FUNCTION FC 101 : VOID
TITLE =
VERSION : 0.1

BEGIN
NETWORK
TITLE =
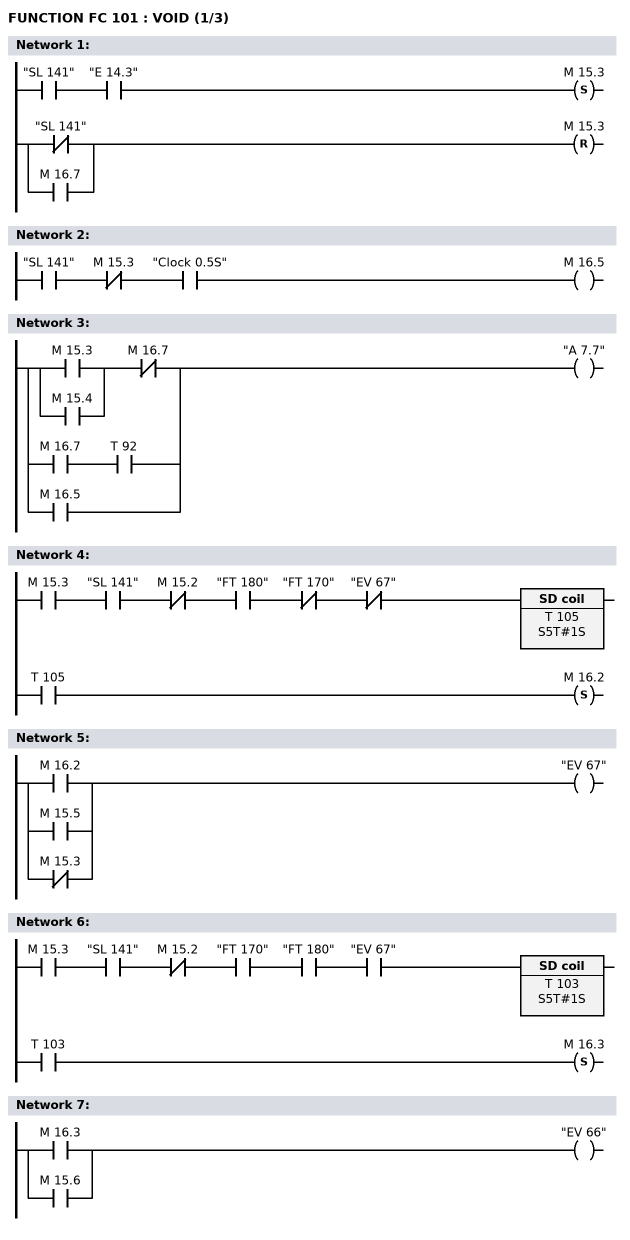
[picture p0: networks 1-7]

      U     "SL 141";
      U     "E      14.3";
      S     M     15.3;
      UN    "SL 141";
      O     M     16.7;
      R     M     15.3;
NETWORK
TITLE =

      U     "SL 141";
      UN    M     15.3;
      U     "Clock 0.5S";
      =     M     16.5;


NETWORK
TITLE =

      U     M     15.3;
      O     M     15.4;
      UN    M     16.7;
      O(    ;
      U     M     16.7;
      U     T     92;
      )     ;
      O     M     16.5;
      =     "A       7.7";
NETWORK
TITLE =

      U     M     15.3;
      U     "SL 141";
      UN    M     15.2;
      U     "FT 180";
      UN    "FT 170";
      UN    "EV 67";
      L     S5T#1S;
      SE    T    105;
      U     T    105;
      S     M     16.2;
NETWORK
TITLE =

      O     M     16.2;
      O     M     15.5;
      ON    M     15.3;
      =     "EV 67";
NETWORK
TITLE =

      U     M     15.3;
      U     "SL 141";
      UN    M     15.2;
      U     "FT 170";
      U     "FT 180";
      U     "EV 67";
      L     S5T#1S;
      SE    T    103;
      U     T    103;
      S     M     16.3;
NETWORK
TITLE =

      O     M     16.3;
      O     M     15.6;
      =     "EV 66";
NETWORK
TITLE =
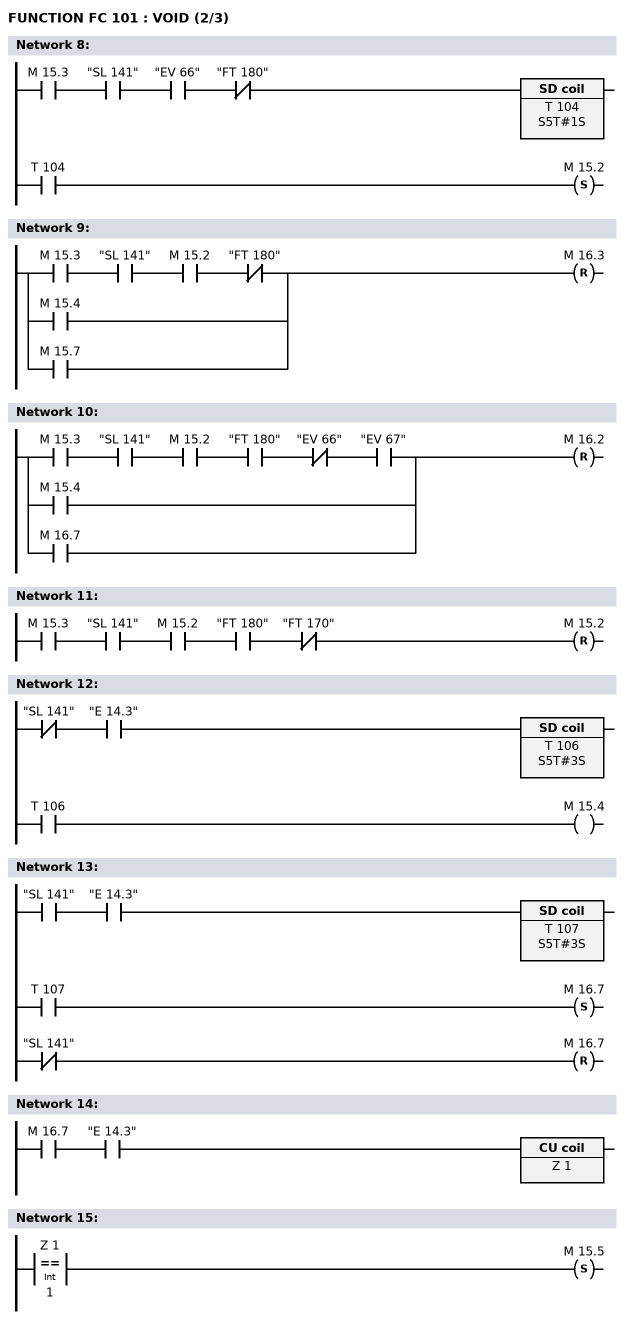
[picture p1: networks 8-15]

      U     M     15.3;
      U     "SL 141";
      U     "EV 66";
      UN    "FT 180";
      L     S5T#1S;
      SE    T    104;
      U     T    104;
      S     M     15.2;
NETWORK
TITLE =

      U     M     15.3;
      U     "SL 141";
      U     M     15.2;
      UN    "FT 180";
      O     M     15.4;
      O     M     15.7;
      R     M     16.3;
NETWORK
TITLE =

      U     M     15.3;
      U     "SL 141";
      U     M     15.2;
      U     "FT 180";
      UN    "EV 66";
      U     "EV 67";
      O     M     15.4;
      O     M     16.7;
      R     M     16.2;
NETWORK
TITLE =

      U     M     15.3;
      U     "SL 141";
      U     M     15.2;
      U     "FT 180";
      UN    "FT 170";
      R     M     15.2;
NETWORK
TITLE =

      UN    "SL 141";
      U     "E      14.3";
      L     S5T#3S;
      SE    T    106;
      U     T    106;
      =     M     15.4;
NETWORK
TITLE =

      U     "SL 141";
      U     "E      14.3";
      L     S5T#3S;
      SE    T    107;
      U     T    107;
      S     M     16.7;
      UN    "SL 141";
      R     M     16.7;
NETWORK
TITLE =

      U     M     16.7;
      U     "E      14.3";
      ZV    Z      1;
NETWORK
TITLE =

      L     Z      1;
      L     1;
      ==I   ;
      S     M     15.5;
NETWORK
TITLE =
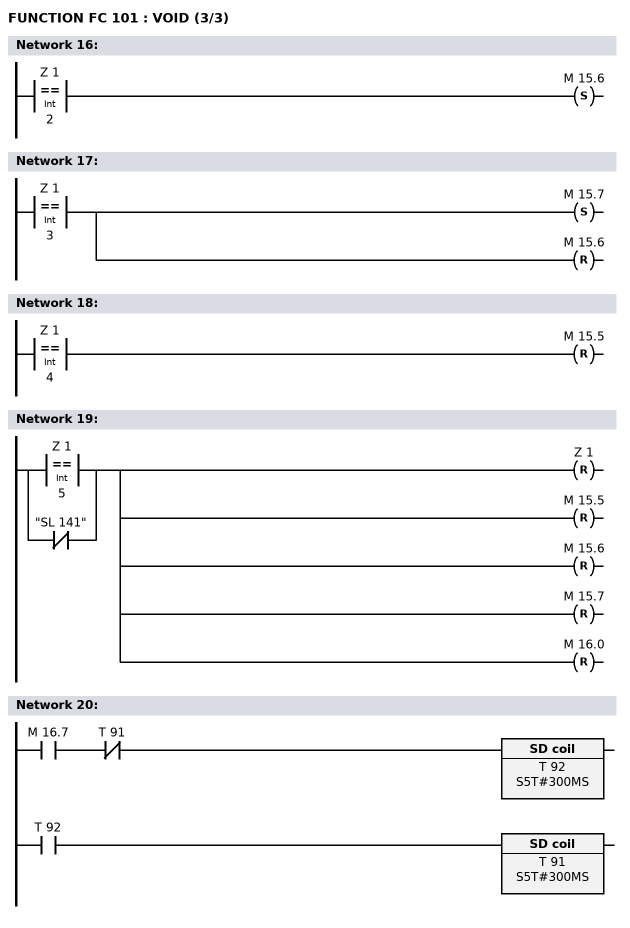
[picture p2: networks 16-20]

      L     Z      1;
      L     2;
      ==I   ;
      S     M     15.6;
NETWORK
TITLE =

      L     Z      1;
      L     3;
      ==I   ;
      S     M     15.7;
      R     M     15.6;
NETWORK
TITLE =

      L     Z      1;
      L     4;
      ==I   ;
      R     M     15.5;
NETWORK
TITLE =

      L     Z      1;
      L     5;
      ==I   ;
      ON    "SL 141";
      R     Z      1;
      R     M     15.5;
      R     M     15.6;
      R     M     15.7;
      R     M     16.0;
NETWORK
TITLE =

      U     M     16.7;
      UN    T     91;
      L     S5T#300MS;
      SE    T     92;
      U     T     92;
      L     S5T#300MS;
      SE    T     91;
END_FUNCTION

